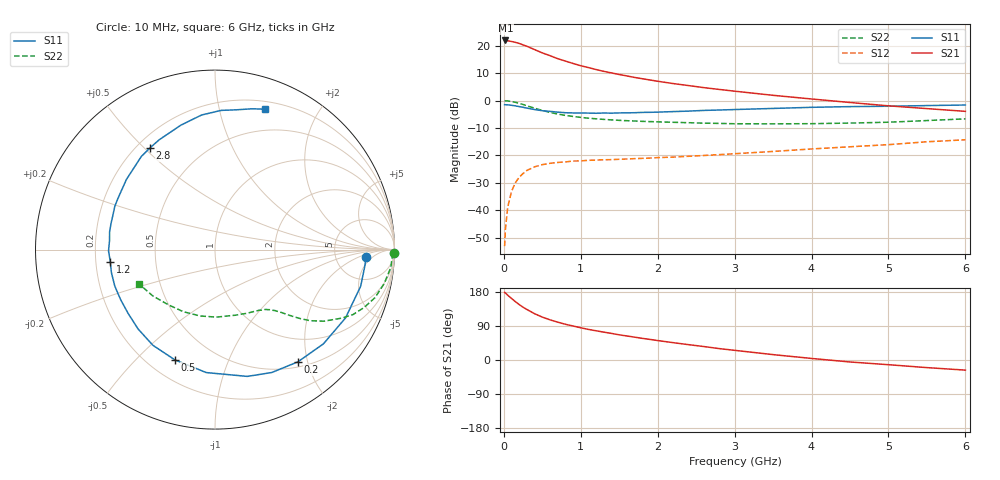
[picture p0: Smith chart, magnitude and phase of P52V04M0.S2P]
! SIEMENS Small Signal Semiconductors
! BFP183
! Si NPN RF Bipolar Junction Transistor in SOT143
! VCE = 2 V  IC = 4 mA
! Common Emitter S-Parameters:  March  1996
# GHz  S  MA  R  50
!  f  S11  S21  S12  S22
! GHz  MAG  ANG  MAG  ANG  MAG  ANG  MAG  ANG
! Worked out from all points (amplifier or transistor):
!   36 points, 10 MHz to 6 GHz, reference 50 ohm
!   highest |S21| = 22.0 dB at 20 MHz (marker M1)
!   |S21| within 3 dB of that: start of sweep to 372 MHz
!   unconditionally stable (mu >= 1): 1.663 GHz to 5.751 GHz
!   at 250 MHz: K = 0.18, MSG = 23.5 dB, |S12| = -26.6 dB
!   at 1.4 GHz: K = 0.89, MSG = 15.8 dB, |S12| = -21.6 dB
!   at 6 GHz: K = 0.96, MSG = 5.2 dB, |S12| = -14.3 dB
!   S11 on the Smith chart (normalised r, x): 10 MHz: 11, -3; 200 MHz: 0.58, -1.84; 500 MHz: 0.31, -0.66; 1.2 GHz: 0.26, -0.05; 2.8 GHz: 0.25, +0.52; 6 GHz: 0.27, +1.38
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0.01  0.8417 -2.8  12.47 178.4  0.0022 90.7  0.9957 -1.2
0.02  0.8403 -5.9  12.52 176.9  0.0044 85.4  0.9886 -2.3
0.05  0.8369 -14.1  12.38 171.1  0.0113 85.1  0.9845 -5.8
0.1  0.8209 -27.6  11.99 162.4  0.022 74.1  0.9613 -11.4
0.15  0.8004 -41.0  11.56 154.0  0.0317 68.2  0.9309 -16.7
0.2  0.7773 -53.6  11.04 146.3  0.0399 62.8  0.8912 -21.2
0.25  0.7543 -65.2  10.39 139.2  0.0467 57.2  0.8499 -25.2
0.3  0.7291 -75.7  9.803 133.3  0.0531 53.0  0.8027 -28.4
0.4  0.6868 -94.1  8.526 122.1  0.0618 45.2  0.7267 -33.3
0.5  0.6537 -110.0  7.42 113.2  0.0677 39.6  0.6613 -36.8
0.6  0.6356 -123.0  6.612 106.0  0.0716 35.7  0.6084 -39.1
0.7  0.6158 -134.1  5.823 99.9  0.0742 32.6  0.5678 -40.8
0.8  0.6005 -143.8  5.267 94.3  0.076 30.2  0.5366 -42.2
1.1  0.5912 -167.5  4.005 80.7  0.0812 26.3  0.4775 -45.4
1.2  0.5873 -173.5  3.684 77.1  0.0821 25.4  0.4651 -46.6
1.7  0.601 160.7  2.645 60.3  0.0872 25.0  0.4241 -52.8
2.2  0.6298 141.5  2.047 45.8  0.093 25.9  0.4016 -60.6
2.8  0.6727 122.5  1.598 30.1  0.1031 27.1  0.3832 -72.5
3.5  0.7191 105.3  1.248 14.2  0.118 27.8  0.3764 -88.8
4.5  0.7763 87.5  0.923 -5.2  0.1435 25.4  0.3885 -117.1
5.5  0.8111 75.3  0.714 -20.1  0.1772 21.3  0.4323 -143.4
6  0.8304 70.4  0.636 -26.7  0.1924 17.4  0.4639 -155.5
